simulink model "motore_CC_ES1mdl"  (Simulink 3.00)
settings: Solver=ode45  StartTime=0.0  StopTime=10.0  RelTol=1e-6  AbsTol=1e-6
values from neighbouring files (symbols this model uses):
  b = 0.8*Nm*s/rad    (= 0.8)    [motore_CC_ES1.m]
  Imax = 5*Amp    (= 5)    [motore_CC_ES1.m]
  J = 1.6*kg*m^2    (= 1.6)    [motore_CC_ES1.m]
  Ke = 8*N*m/Amp    (= 8)    [motore_CC_ES1.m]
  L = 0.1*Henry    (= 0.1)    [motore_CC_ES1.m]
  R = 8*Ohm    (= 8)    [motore_CC_ES1.m]
libraries: cstblocks x3

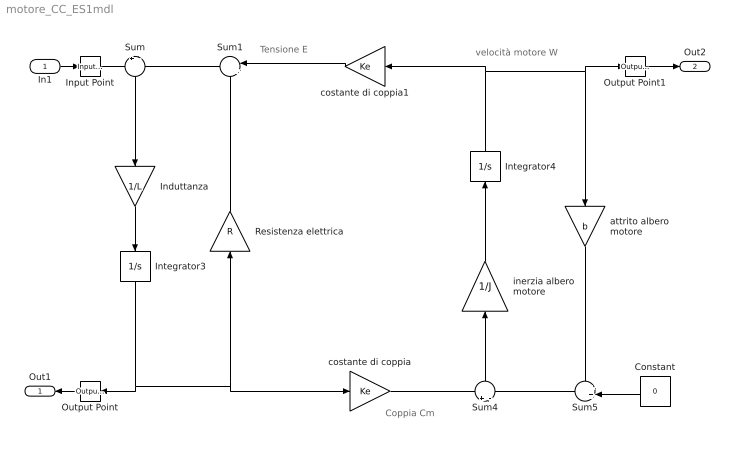
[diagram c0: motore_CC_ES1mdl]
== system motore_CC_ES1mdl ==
  note: Tensione E
  note: velocità motore W
  note: Coppia Cm
  In1 : Inport  Port=1  PortWidth=-1  SampleTime=-1  DataType=auto
  Constant : Constant  Orientation=left  Value=0
  Induttanza : Gain  Orientation=down  Gain=1/L  SaturateOnIntegerOverflow=on
  Input Point : cstblocks/Input Point  PerturbationValue=0
  Integrator3 : Integrator  Orientation=down  ExternalReset=none  InitialConditionSource=internal  InitialCondition=0  LimitOutput=on  UpperSaturationLimit=Imax  LowerSaturationLimit=-Imax  ShowSaturationPort=off  ShowStatePort=off  AbsoluteTolerance=auto
  Integrator4 : Integrator  Orientation=up  ExternalReset=none  InitialConditionSource=internal  InitialCondition=0  LimitOutput=off  UpperSaturationLimit=inf  LowerSaturationLimit=-inf  ShowSaturationPort=off  ShowStatePort=off  AbsoluteTolerance=auto
  Output Point : cstblocks/Output Point  Orientation=left  SigprobeOutputIndex=1
  Output Point1 : cstblocks/Output Point  SigprobeOutputIndex=2
  Resistenza elettrica : Gain  Orientation=up  Gain=R  SaturateOnIntegerOverflow=on
  Sum : Sum  Orientation=down  Inputs=+|-  SaturateOnIntegerOverflow=on
  Sum1 : Sum  Orientation=left  Inputs=|++  SaturateOnIntegerOverflow=on
  Sum4 : Sum  Orientation=up  Inputs=+|-  SaturateOnIntegerOverflow=on
  Sum5 : Sum  Orientation=left  Inputs=++|  SaturateOnIntegerOverflow=on
  attrito albero motore : Gain  Orientation=down  Gain=b  SaturateOnIntegerOverflow=on
  costante di coppia : Gain  Gain=Ke  SaturateOnIntegerOverflow=on
  costante di coppia1 : Gain  Orientation=left  Gain=Ke  SaturateOnIntegerOverflow=on
  inerzia albero motore : Gain  Orientation=up  Gain=1/J  SaturateOnIntegerOverflow=on
  Out1 : Outport  Orientation=left  Port=1
  Out2 : Outport  Port=2
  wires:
  Sum/1 -> Induttanza/1
  Induttanza/1 -> Integrator3/1
  Sum1/1 -> Sum/2
  Resistenza elettrica/1 -> Sum1/2
  Sum4/1 -> inerzia albero motore/1
  inerzia albero motore/1 -> Integrator4/1
  Sum5/1 -> Sum4/2
  attrito albero motore/1 -> Sum5/1
  Integrator4/1 -> costante di coppia1/1, attrito albero motore/1, Output Point1/1
  costante di coppia1/1 -> Sum1/1
  Constant/1 -> Sum5/2
  costante di coppia/1 -> Sum4/1
  Integrator3/1 -> Resistenza elettrica/1, costante di coppia/1, Output Point/1
  In1/1 -> Input Point/1
  Input Point/1 -> Sum/1
  Output Point/1 -> Out1/1
  Output Point1/1 -> Out2/1
